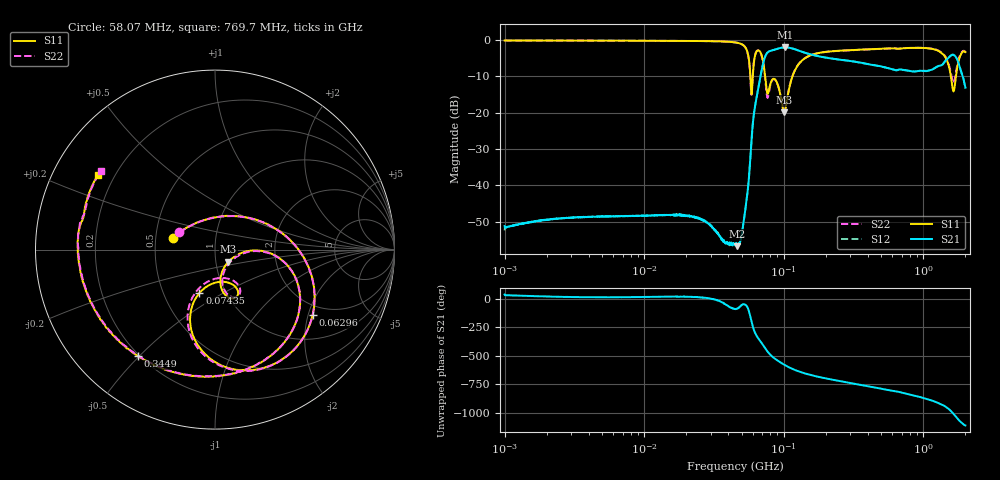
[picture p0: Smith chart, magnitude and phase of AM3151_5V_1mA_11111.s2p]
! Date/Time: Fri Jun 26 11:17:45 2020
! Network Analyzer:  Rev:
! Sweep from 1000000.0 to 2000000000.0, 1601 Points ! Power Supply: 0 V, 0 A
# HZ S DB R 50
!freq MagS11 AngS11 MagS21 AngS21 MagS12 AngS12 MagS22 AngS22
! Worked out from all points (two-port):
!   1601 points, 1 MHz to 2 GHz, reference 50 ohm
!   highest |S21| = -2.03 dB at 102.2 MHz (marker M1); lowest = -56.7 dB at 46.23 MHz (marker M2)
!   |S21| within 3 dB of the highest: 72.86 MHz to 213 MHz (140.2 MHz wide, 98.1 % of centre); 1.505 GHz to 1.73 GHz (224.5 MHz wide, 13.9 % of centre)
!   lowest |S11| = -19.9 dB at 100.8 MHz (marker M3), VSWR 1.22, Z = 57.5 - j7.88 ohm
!   |S11| at or under -10 dB: 57.65 MHz to 59.98 MHz (2.326 MHz wide, 3.95 % of centre); 73.5 MHz to 115.4 MHz (41.88 MHz wide, 44.3 % of centre); 1.574 GHz to 1.711 GHz (137.6 MHz wide, 8.38 % of centre)
!   |S22| runs from -19.2 to -0.2 dB; largest |S21 - S12| = 0.0081
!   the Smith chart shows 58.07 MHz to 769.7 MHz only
!   S11 on the Smith chart (normalised r, x): 58.07 MHz: 0.61, +0.09; 62.96 MHz: 1.67, -2.14; 74.35 MHz: 0.75, -0.39; 344.9 MHz: 0.19, -0.50; 769.7 MHz: 0.14, +0.28
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1000000  -0.16 -1.4  -51.16 38.8  -52.39 36.8  -0.16 -1.4
3555161  -0.20 -4.3  -48.67 16.0  -48.73 15.2  -0.19 -4.3
1.263916e7  -0.26 -14.7  -48.14 19.6  -48.21 19.3  -0.25 -14.7
4.493426e7  -0.70 -65.6  -56.33 -87.5  -56.41 -86.4  -0.70 -65.8
4.623347e7  -0.77 -69.3  -56.69 -85.7  -56.28 -84.4  -0.78 -69.6
5.281102e7  -1.94 -99.6  -47.12 -48.5  -47.04 -48.9  -1.99 -100.5
5.807476e7  -12.20 164.1  -30.28 -173.1  -30.27 -173.2  -13.12 154.3
6.295945e7  -3.67 -33.9  -17.08 50.3  -17.09 50.3  -3.54 -36.2
6.760948e7  -3.26 -78.0  -10.62 -7.4  -10.62 -7.4  -3.29 -79.8
7.434822e7  -11.79 -109.8  -4.16 -81.2  -4.16 -81.2  -12.45 -112.9
8.533003e7  -10.71 -69.2  -2.72 -159.3  -2.73 -159.3  -10.78 -66.2
1.007655e8  -19.92 -42.2  -2.04 142.7  -2.03 142.6  -19.24 -40.6
1.022118e8  -19.44 -27.5  -2.03 138.3  -2.03 138.3  -18.77 -27.1
1.589914e8  -4.09 -46.4  -4.07 49.8  -4.07 49.7  -4.10 -46.6
3.448783e8  -2.70 -125.8  -6.15 -31.7  -6.18 -31.6  -2.73 -126.5
5.652395e8  -2.35 -177.0  -7.82 -80.7  -7.79 -80.6  -2.36 -178.8
7.69728e8  -2.23 147.7  -8.43 -114.1  -8.41 -113.8  -2.24 145.2
1.152667e9  -2.47 87.1  -8.16 -171.9  -8.12 -171.8  -2.41 84.7
1.413901e9  -4.33 42.3  -6.07 141.3  -6.04 141.3  -4.22 42.6
1.592202e9  -11.28 20.1  -4.17 90.3  -4.14 90.4  -10.04 24.7
1.750899e9  -7.44 71.0  -5.43 31.1  -5.44 30.7  -6.79 62.4
2e9  -3.35 15.0  -13.11 -30.4  -13.28 -31.1  -3.43 10.4
